TYPE Meter_Data :
STRUCT
	AlmEn_In_b			    :	BOOL;//使能
	OverRangeAlm_In_b	    :	BOOL;//超上限报警
	UnderRangeAlm_In_b	    :	BOOL;//超下限报警
	AlmRst_In_b			    :	BOOL;//报警复位
	AnalogRdValue_In_Int	:	INT;//实际通道值
	AnalogResMax_In_Int	    :	INT;//通道最大值
	AnalogResMin_In_Int   	:	INT;//通道最小值
	AnalogPhyMax_In_Real	:	REAL;//工程量最大值
	AnalogPhyMin_In_Real	:	REAL;//工程量最小值
    AlmDnLmtSV_In_Real	    :	REAL;//设定最小值
	AlmUpLmtSV_In_Real	    :	REAL;//设定最大值
	AnalogRdOffset_In_Real	:	REAL;//偏移值
	
	ActRdValue_Out_Real	        :	REAL;
	ActValueOutRangeAlm_Out_b	:	BOOL;
	ActValueStatusOK_Out_b	    :	BOOL;
END_STRUCT
END_TYPE
